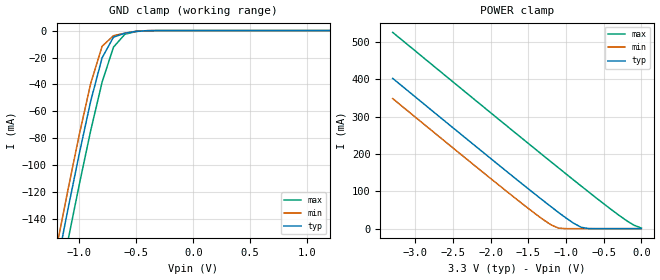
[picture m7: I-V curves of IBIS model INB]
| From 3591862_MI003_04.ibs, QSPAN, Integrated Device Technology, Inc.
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|   Model INB
[Model]   INB
Model_type   Input
Polarity   Non-Inverting
Vinl =   0.8000V
Vinh =   2.0000V
C_comp   5.00pF   5.00pF   5.00pF
[Voltage Range]   3.3000V   3.0000V   4.0000V
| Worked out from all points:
|   GND clamp passes 1 mA (typ) near -0.53 V on its own axis
|   POWER clamp passes 1 mA (typ) near -0.72 V on its own axis
[GND_clamp]
| voltage   I(typ)   I(min)   I(max)
-3.3V     -1.129A    -1.116A    -1.151A
-1.2V     -175.8mA   -161.3mA   -199.1mA
-1.1V     -132.8mA   -118.4mA   -156.1mA
-1V       -91.26mA   -77.09mA   -114.2mA
-900mV    -52.33mA   -39.25mA   -74.22mA
-800mV    -20.19mA   -11.67mA   -38.26mA
-700mV    -4.874mA   -3.78mA    -12.27mA
-600mV    -1.934mA   -1.91mA    -2.712mA
-500mV    -558.6uA   -499.9uA   -686uA
-400mV    -63.12uA   -39.91uA   -111.1uA
1.2V      10.39pA    3.135pA    188.9pA
[POWER_clamp]
| voltage   I(typ)   I(min)   I(max)
-3.3V     402.4mA    348.3mA    525.5mA
-1.8V     155.3mA    101.9mA    277.5mA
-1.4V     90.64mA    38.72mA    211.8mA
-1.2V     59mA       10.41mA    179.2mA
-1.1V     43.57mA    1.444mA    162.9mA
-900mV    14.76mA    424.9nA    130.5mA
-800mV    3.845mA    6.094nA    114.4mA
-700mV    187.3uA    108.3pA    98.4mA
-200mV    32pA       17.95pA    22.07mA
-100mV    30.48pA    17.27pA    9.496mA
0V        29.78pA    16.6pA     1.592mA
